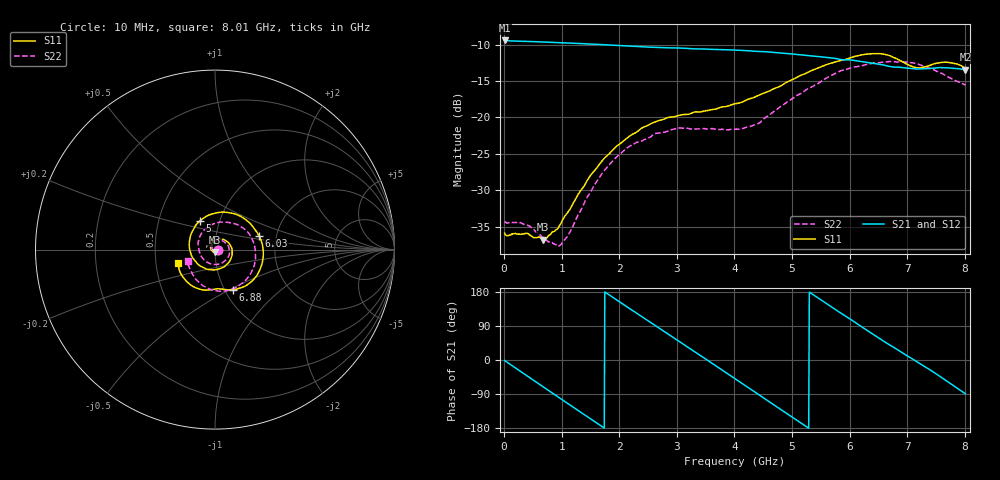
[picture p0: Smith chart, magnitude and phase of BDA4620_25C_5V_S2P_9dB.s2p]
!Agilent Technologies,E5071B,MY42404982,A.09.10
!Date: Wed May 06 09:00:02 2026
!Data & Calibration Information:
!Freq	S11:SOLT2(ON)	S21:SOLT2(ON)	S12:SOLT2(ON)	S22:SOLT2(ON)
# Hz S RI R 50
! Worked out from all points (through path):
!   801 points, 10 MHz to 8.01 GHz, reference 50 ohm
!   highest |S21| = -9.45 dB at 10 MHz (marker M1); lowest = -13.5 dB at 8.01 GHz (marker M2)
!   group delay of S21, straight-line fit = 280 ps
!   lowest |S11| = -36.8 dB at 680 MHz (marker M3), VSWR 1.03, Z = 49.9 - j1.44 ohm
!   |S11| at or under -10 dB: start of sweep to end of sweep
!   |S22| runs from -37.6 to -12.3 dB; largest |S21 - S12| = 0.0015
!   S11 on the Smith chart (normalised r, x): 10 MHz: 1.03, -0.00; 5 GHz: 0.81, +0.27; 6.03 GHz: 1.63, +0.26; 6.88 GHz: 1.10, -0.52; 8.01 GHz: 0.65, -0.10
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1e7  0.0161 -0.00115  0.337 -0.00724  0.3375 -0.00717  0.0194 -0.00118
3.2e8  0.0126 -0.00964  0.2772 -0.184  0.2775 -0.1842  0.0164 -0.00903
6.8e8  -0.001 -0.0145  0.1081 -0.3107  0.1079 -0.3114  0.00381 -0.0145
9.8e8  -0.0175 -0.00632  -0.0662 -0.3187  -0.0666 -0.3192  -0.0107 -0.0081
1.35e9  -0.0246 0.021  -0.2447 -0.2071  -0.245 -0.2074  -0.0185 0.015
1.65e9  -0.01 0.0463  -0.3117 -0.0531  -0.3123 -0.0532  -0.00886 0.0374
1.94e9  0.0196 0.0596  -0.2937 0.1059  -0.2943 0.1063  0.015 0.0509
2.32e9  0.0661 0.0459  -0.1602 0.2617  -0.1606 0.2621  0.0533 0.0421
2.68e9  0.095 0.000654  0.0241 0.3011  0.0246 0.3015  0.0774 0.0106
3e9  0.0872 -0.0535  0.1797 0.2396  0.1801 0.2398  0.0789 -0.0294
3.39e9  0.0363 -0.1028  0.2866 0.0704  0.2871 0.0701  0.0434 -0.0712
4.01e9  -0.0899 -0.0853  0.1886 -0.2195  0.1887 -0.2202  -0.0549 -0.0625
4.49e9  -0.1437 0.0242  -0.0411 -0.2801  -0.0413 -0.2805  -0.0936 0.0221
5e9  -0.0823 0.1614  -0.2371 -0.1342  -0.2376 -0.1341  -0.0357 0.1294
5.35e9  0.0306 0.2083  -0.2622 0.0274  -0.2625 0.0274  0.0558 0.1524
6.03e9  0.2462 0.0757  -0.0674 0.238  -0.0673 0.2385  0.2157 0.0371
6.36e9  0.2634 -0.0716  0.0712 0.2259  0.0714 0.2261  0.2228 -0.0689
6.68e9  0.18 -0.1964  0.1689 0.1472  0.1694 0.1475  0.1756 -0.1656
6.88e9  0.1015 -0.2235  0.2039 0.0844  0.2045 0.0847  0.1232 -0.2071
7.19e9  0.0168 -0.218  0.2133 -0.0242  0.214 -0.0244  0.0169 -0.2314
7.55e9  -0.0902 -0.2185  0.1648 -0.1453  0.1647 -0.1454  -0.088 -0.1837
8.01e9  -0.2047 -0.0729  0.00325 -0.2121  0.0035 -0.2127  -0.1524 -0.0661
